FUNCTION FC 100 : VOID
TITLE =BLOCK FOR START/STOP TORC PAC
AUTHOR : Esposito
FAMILY : EGAL_srl
NAME : TORC_PAC
VERSION : 0.1

BEGIN
NETWORK
TITLE =CONDITIONS FOR START/STOP TORC PAC
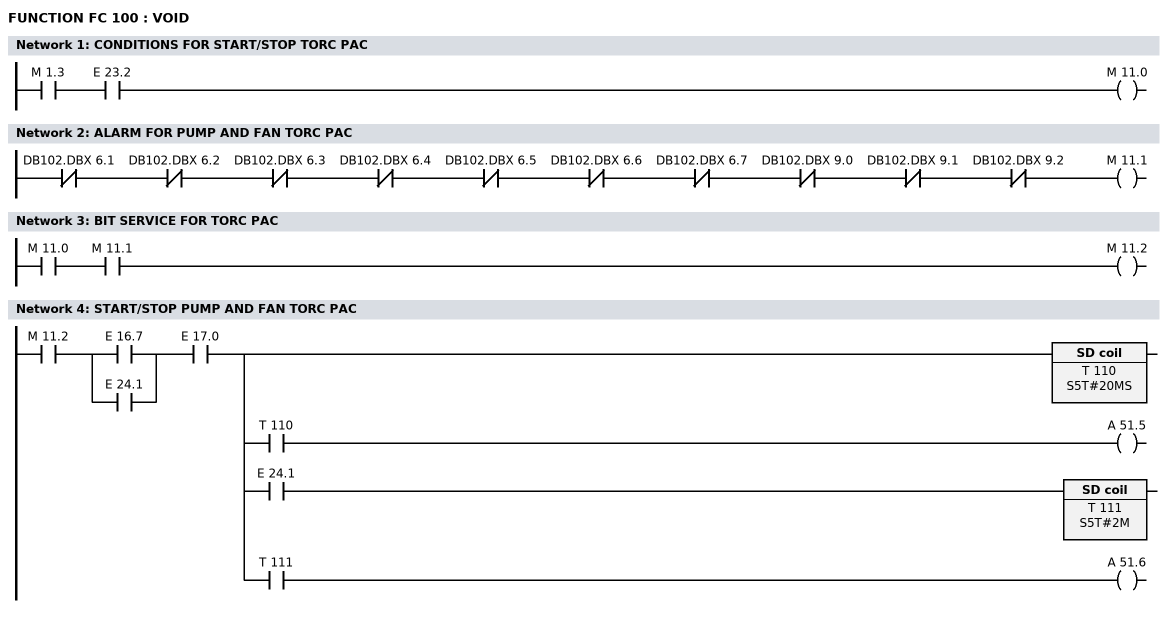
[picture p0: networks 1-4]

      U     M      1.3;
      U     E     23.2;
      =     M     11.0;
NETWORK
TITLE =ALARM FOR PUMP AND FAN TORC PAC

      UN    DB102.DBX    6.1;
      UN    DB102.DBX    6.2;
      UN    DB102.DBX    6.3;
      UN    DB102.DBX    6.4;
      UN    DB102.DBX    6.5;
      UN    DB102.DBX    6.6;
      UN    DB102.DBX    6.7;
      UN    DB102.DBX    9.0;
      UN    DB102.DBX    9.1;
      UN    DB102.DBX    9.2;
      =     M     11.1;
NETWORK
TITLE =BIT SERVICE FOR TORC PAC

      U     M     11.0;
      U     M     11.1;
      =     M     11.2;
NETWORK
TITLE =START/STOP PUMP AND FAN TORC PAC

      U     M     11.2;
      U(    ;
      O     E     16.7;
      O     E     24.1;
      )     ;
      U     E     17.0;
      =     L      0.0;
      U     L      0.0;
      BLD   102;
      L     S5T#20MS;
      SE    T    110;
      U     L      0.0;
      U     T    110;
      =     A     51.5;
      U     L      0.0;
      U     E     24.1;
      L     S5T#2M;
      SE    T    111;
      U     L      0.0;
      U     T    111;
      =     A     51.6;
END_FUNCTION

